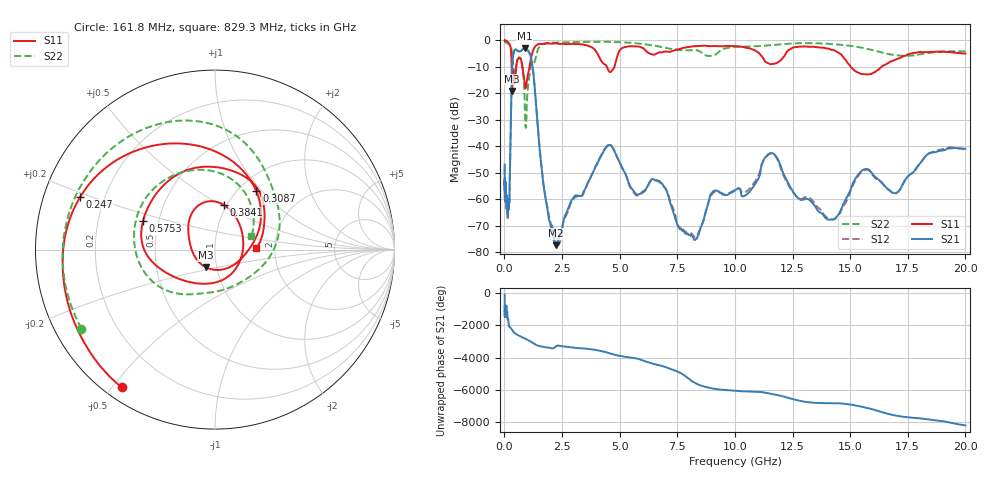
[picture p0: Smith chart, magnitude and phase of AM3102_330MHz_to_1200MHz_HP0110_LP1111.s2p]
! Date/Time: Tue, Sep 11, 2018 5:15 PM
! Network Analyzer: Agilent Technologies E8362B Rev: A.07.50.63
! Sweep from 0.010 to 20.000 GHz, 1601 Points, Sweep Type: LOG
! Power Supply: 4.949 V, 0.001 A
# Hz S DB R 50
!freq MagS11 AngS11 MagS21 AngS21 MagS12 AngS12 MagS22 AngS22
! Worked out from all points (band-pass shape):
!   1601 points, 10 MHz to 20 GHz, reference 50 ohm
!   highest |S21| = -3.05 dB at 890.6 MHz (marker M1); lowest = -77.4 dB at 2.228 GHz (marker M2)
!   |S21| within 3 dB of the highest: 372.1 MHz to 1.139 GHz (766.6 MHz wide, 101 % of centre)
!   lowest |S11| = -19.1 dB at 337.9 MHz (marker M3), VSWR 1.25, Z = 44.3 - j8.85 ohm
!   |S11| at or under -10 dB: 780 MHz to 1.089 GHz (309.1 MHz wide, 33.1 % of centre); 4.444 GHz to 4.77 GHz (326.1 MHz wide, 7.08 % of centre); 15.03 GHz to 16.37 GHz (1.343 GHz wide, 8.56 % of centre)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
!   |S22| runs from -33.1 to -0.3 dB; largest |S21 - S12| = 0.012
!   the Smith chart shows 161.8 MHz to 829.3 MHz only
!   S11 on the Smith chart (normalised r, x): 161.8 MHz: 0.05, -0.53; 247 MHz: 0.11, +0.19; 308.7 MHz: 1.21, +0.93; 384.1 MHz: 0.97, +0.52; 575.3 MHz: 0.41, +0.16; 829.3 MHz: 1.59, +0.03
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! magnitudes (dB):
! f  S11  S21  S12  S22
! 10 MHz  0.0  -46.9  -47.7  -0.3
! 35.55 MHz  0.0  -57.6  -56.3  -0.6
! 126.4 MHz  -0.4  -62.7  -64.3  -1.1
! 161.8 MHz  -0.7  -66.8  -63.0  -1.3
! 247 MHz  -1.9  -46.5  -46.8  -1.7
! 308.7 MHz  -8.0  -17.9  -18.0  -3.3
! 337.9 MHz  -19.1  -9.6  -9.6  -5.7
! 384.1 MHz  -11.9  -5.4  -5.5  -9.4
! 447.2 MHz  -15.7  -3.6  -3.7  -12.8
! 575.3 MHz  -7.3  -4.0  -4.0  -7.1
! 829.3 MHz  -12.8  -3.2  -3.2  -13.3
! 890.6 MHz  -17.1  -3.1  -3.1  -27.3
! 1.219 GHz  -4.5  -9.7  -9.7  -8.3
! 1.59 GHz  -1.4  -46.2  -46.1  -1.8
! 2.228 GHz  -1.1  -77.4  -76.6  -0.8
! 4.479 GHz  -10.7  -39.9  -39.7  -0.5
! 5.652 GHz  -2.2  -57.5  -57.9  -1.0
! 6.739 GHz  -4.5  -53.4  -53.7  -2.4
! 8.149 GHz  -2.3  -73.9  -73.3  -3.7
! 11.53 GHz  -9.0  -42.6  -42.9  -1.8
! 14.07 GHz  -3.2  -67.8  -67.3  -1.3
! 20 GHz  -4.9  -41.0  -41.3  -4.2
